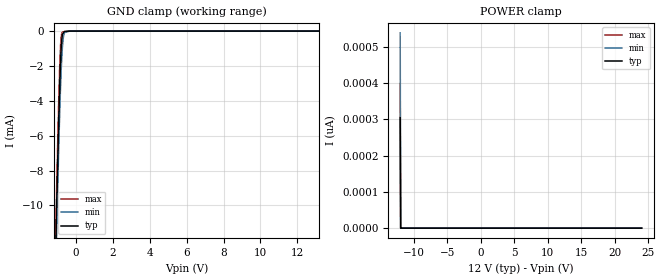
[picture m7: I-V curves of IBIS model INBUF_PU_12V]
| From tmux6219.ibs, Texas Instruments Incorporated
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| Model8
[Model]   INBUF_PU_12V
Model_type   Input
Vinl = 0.8
Vinh = 1.3
|   typ   min   max
C_comp   1.85pF   1.7pF   2.1pF
[Voltage Range]   12   10.8   13.2
[Temperature Range]   27   125   -40
[Power Clamp Reference]   12   10.8   13.2
[GND Clamp Reference]   0   0   0
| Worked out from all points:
|   GND clamp passes 1 mA (typ) near -0.80 V on its own axis
[GND Clamp]
|   Voltage   I(typ)   I(min)   I(max)
-12V      -596.9mA   -596.1mA   -597.6mA
-1.128V   -14.01mA   -15.32mA   -12.97mA
-1.092V   -12.28mA   -13.63mA   -11.2mA
-1.056V   -10.57mA   -11.97mA   -9.464mA
-1.02V    -8.907mA   -10.35mA   -7.765mA
-912mV    -4.294mA   -5.832mA   -3.1mA
-840mV    -1.878mA   -3.32mA    -895.7uA
-804mV    -1.033mA   -2.308mA   -336.7uA
-732mV    -184uA     -882.7uA   -63.06uA
-696mV    -130.3uA   -461.1uA   -52.53uA
-624mV    -22.84uA   -88.74uA   -31.47uA
24V       0A         0A         0A
[POWER Clamp]
|   Voltage   I(typ)   I(min)   I(max)
-12V      304.1pA    537.7pA    397.9pA
-11.93V   0A         0A         0A
-11.89V   0A         0A         0A
24V       0A         0A         0A
